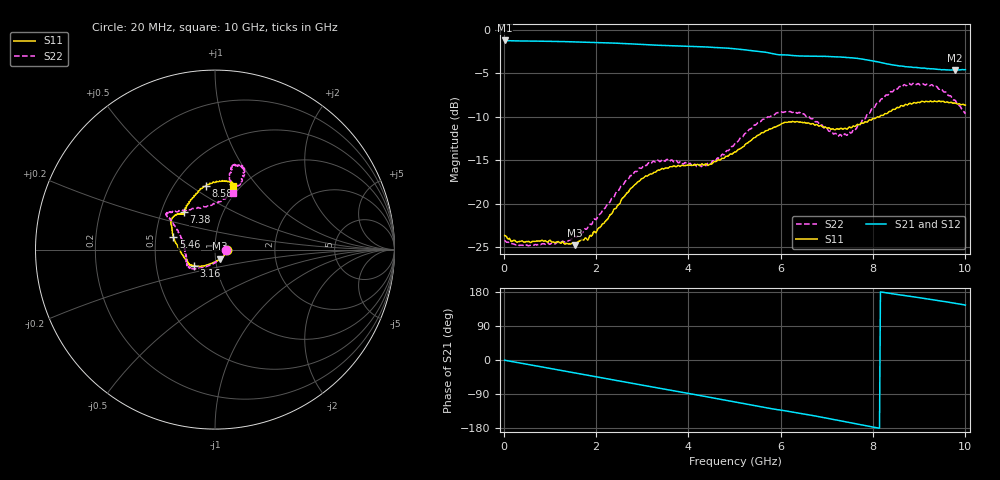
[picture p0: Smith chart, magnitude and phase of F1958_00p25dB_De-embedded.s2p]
! Integrated Device Technology
! Corporate Headquarters
! 6024 Silver Creek Valley Road
! San Jose, CA 95138  USA
! Phone:  1-408-284-8200
! Toll Free:  1-800-223-1366
! Webpage:  http://www.idt.com/
! Timing and RF Division
! 515 Groton Road, Suite 102
! Westford, MA 01886-6024
! Device:  F1958
! Description: 7-bit 0.25 dB Digital Step Attenuator
! Frequency:  0.001 -  6.000 GHz
! Package:  4x4 mm Thin QFN Plastic Package: 24 pin
! Ports:  2 RF, 12 DC
!  Pin  1  = D0
!  Pin  2  = VDD
!  Pin  3  = VMODE
!  Pin  4  = GND
!  Pin  5  = RF1  =  Port 1
!  Pin  6  = GND
!  Pin  7  = GND
!  Pin  8  = GND
!  Pin  9  = GND
!  Pin 10  = GND
!  Pin 11  = GND
!  Pin 12  = GND
!  Pin 13  = GND
!  Pin 14  = RF2  =  Port 2
!  Pin 15  = GND
!  Pin 16  = LE
!  Pin 17  = CLK
!  Pin 18  = DATA
!  Pin 19  = D6
!  Pin 20  = D5
!  Pin 21  = D4
!  Pin 22  = D3
!  Pin 23  = D2
!  Pin 24  = D1
! State:  1
! Atten State:  0.25 dB
! Voltage:  +3.30 Volts
! Current:  0.257 mA
! Data:  The device was measured on a F1958 evaluation board which has
!  individual transmission lines to the RF pins.  Data was collected
!  using a calibrated network analyzer.  The evaluation board was
!  de-embedded using Automatic Fixture Removal (AFR).
!  The reference plane is the edge of the package pin.
! Misc:
!  Action Tracker AT0419
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# GHz S dB R 50
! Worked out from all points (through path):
!   500 points, 20 MHz to 10 GHz, reference 50 ohm
!   highest |S21| = -1.25 dB at 20 MHz (marker M1); lowest = -4.7 dB at 9.78 GHz (marker M2)
!   group delay of S21, straight-line fit = 60.4 ps
!   lowest |S11| = -24.7 dB at 1.54 GHz (marker M3), VSWR 1.12, Z = 52.7 - j5.3 ohm
!   |S11| at or under -10 dB: start of sweep to 8.142 GHz
!   |S22| runs from -24.8 to -6.2 dB; largest |S21 - S12| = 0.0022
!   S11 on the Smith chart (normalised r, x): 20 MHz: 1.14, -0.01; 3.16 GHz: 0.78, -0.14; 5.46 GHz: 0.62, +0.09; 7.38 GHz: 0.65, +0.29; 8.58 GHz: 0.71, +0.58; 10 GHz: 0.92, +0.76
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0.02  -23.63 -2.3  -1.25 -0.6  -1.25 -0.6  -24.18 -2.7
0.3  -24.39 -7.1  -1.31 -6.8  -1.31 -6.8  -24.60 -10.6
0.8  -24.24 -19.6  -1.34 -17.7  -1.34 -17.7  -24.69 -26.4
1.54  -24.74 -59.8  -1.42 -34.1  -1.41 -34.1  -23.78 -72.9
1.7  -24.07 -70.4  -1.44 -37.5  -1.43 -37.5  -23.35 -83.5
2.04  -22.88 -94.2  -1.49 -45.1  -1.48 -45.1  -21.44 -103.7
2.72  -18.48 -129.5  -1.63 -60.2  -1.62 -60.2  -16.98 -132.3
3.16  -16.59 -142.6  -1.76 -69.9  -1.75 -70.0  -15.32 -141.9
3.36  -16.13 -145.1  -1.81 -74.2  -1.81 -74.3  -15.06 -145.7
4.34  -15.53 -158.7  -1.99 -95.6  -2.00 -95.7  -15.43 -176.9
5.02  -14.05 179.7  -2.21 -111.0  -2.22 -111.0  -12.97 154.9
5.46  -12.33 163.0  -2.47 -120.9  -2.49 -120.9  -10.94 147.4
5.98  -10.95 149.8  -2.90 -131.7  -2.91 -131.7  -9.47 143.9
6.68  -10.79 136.3  -3.06 -146.2  -3.08 -146.1  -10.23 135.9
7.2  -11.42 131.6  -3.14 -158.0  -3.15 -157.9  -11.94 111.9
7.38  -11.32 129.6  -3.18 -162.4  -3.19 -162.3  -11.99 98.6
7.9  -10.45 118.6  -3.50 -174.7  -3.50 -174.7  -9.61 74.4
8.34  -9.44 106.2  -3.97 176.2  -3.97 176.1  -7.41 68.3
8.58  -8.87 97.7  -4.18 171.9  -4.19 172.0  -6.52 70.1
9.26  -8.23 80.1  -4.50 159.5  -4.51 159.5  -6.34 77.0
9.78  -8.42 74.4  -4.65 149.7  -4.67 149.7  -8.13 77.3
10  -8.68 74.5  -4.59 144.7  -4.62 144.8  -9.66 72.4
